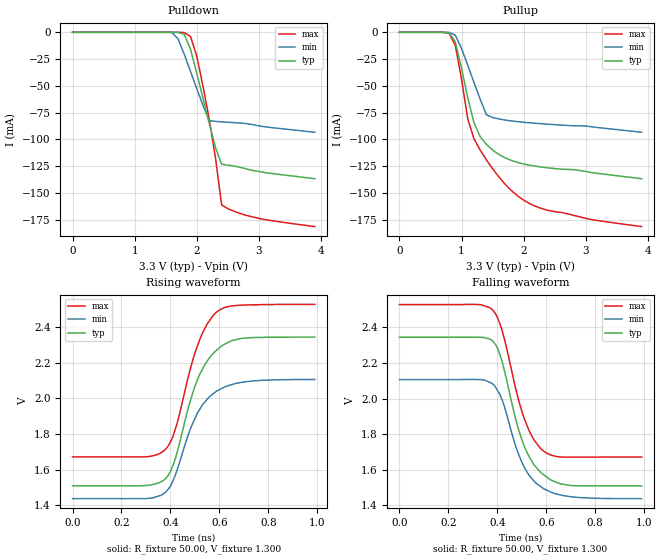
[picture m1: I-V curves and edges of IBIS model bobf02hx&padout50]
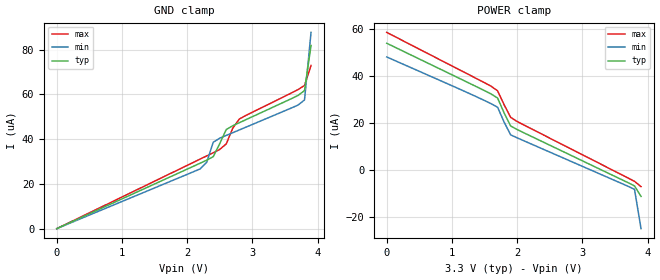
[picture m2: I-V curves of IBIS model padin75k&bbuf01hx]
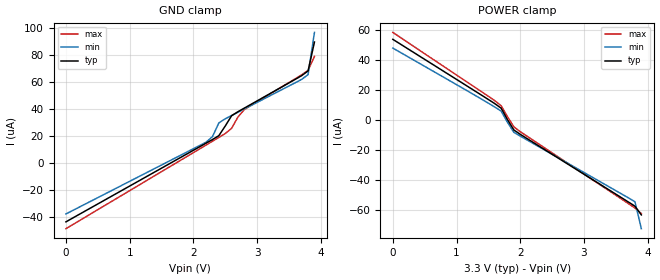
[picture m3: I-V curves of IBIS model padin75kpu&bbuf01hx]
|   This file is an IBIS representation of the   |
|   Integrated Device Technology, Inc.   |
|   MC100ES6254   |
|   2x2 Clock Switch   |
[IBIS Ver]   3.2
[File name]   mc100es6254_3v3.ibs
[File Rev]   0.02
[Date]   7 March 2006 | Last modified
|   7 March 2006 | Generated
[Source]   Originated at Integrated Device Technology, Inc.
[Disclaimer]
   (C) Copyright Integrated Device Technology, Inc. 2005
   All rights reserved
   IDT hereby grants the user of this IBIS model a non-exclusive,
   nontransferable license to use this IBIS model under the following terms.
   Before using this IBIS model, the user should read this license.
   If the user does not accept these terms,  the IBIS model should be
   returned to IDT within 30 days.
   The user is granted this license only to use the IBIS model and
   is not granted rights to sell, load, rent, lease or license the IBIS
   model in whole or in part, or in modified form to anyone other than
   user. User may modify the IBIS model to suit its specific
   applications but rights to derivative works and such modifications
   shall belong to IDT.
   This IBIS model is provided on an "AS IS" basis and IDT makes
   absolutely no warranty with respect to the information contained
   herein. IDT DISCLAIMS AND CUSTOMER WAIVES ALL WARRANTIES, EXPRESS
   OR IMPLIED, INCLUDING WARRANTIES OF MERCHANTABILITY OR FITNESS FOR
   A PARTICULAR PURPOSE. The entire risk as to quality and performance
   is with the Customer. ACCORDINGLY, IN NO EVENT SHALL THE COMPANY BE
   LIABLE FOR ANY DAMAGES, WHETHER IN CONTRACT OR TORT,INCLUDING ANY
   LOST PROFITS OR OTHER INCIDENTAL, CONSEQUENTIAL, EXEMPLARY, OR
   PUNITIVE DAMAGES ARISING OUT OF THE USE OR APPLICATION OF THE IBIS
   model provided in this package. Further, IDT reserves the right to
   make changes without notice to any product herein to improve
   reliability, function, or design. IDT does not convey any license
   under patent rights or any other intellectual property rights,
   including those of third parties.
   IDT is not obligated to provide maintenance or support
   for the licensed IBIS model.
[Copyright]   Copyright 2002 by Integrated Device Technology, Inc.
[Component]   32ld_LQFP
[Manufacturer]   Integrated Device Technology, Inc.
[Package]
   |LQFP32
   |   typ   min   max
   R_pkg   220.4m   212.5m   238m
   L_pkg   1.841n   1.708n   1.974n
   C_pkg   0.316p   0.2907p   0.33p
[Pin]   signal_name   model_name
   1   VCC   POWER
   2   GND   GND
   3   SEL1   padin75k&bc2p01ll
   4   CLK1   padin75k&bbuf01hx
   5   nCLK1   padin75kpu&bbuf01hx
   6   OEB   padin75k&bc2p01ll
   7   GND   GND
   8   VCC   POWER
   9   nQB0   bobf02hx&padout50
   10   QB0   bobf02hx&padout50
   11   VCC   POWER
   12   nQB1   bobf02hx&padout50
   13   QB1   bobf02hx&padout50
   14   VCC   POWER
   15   nQB2   bobf02hx&padout50
   16   QB2   bobf02hx&padout50
   17   VCC   POWER
   18   GND   GND
   19   SEL0   padin75k&bc2p01ll
   20   nCLK0   padin75kpu&bbuf01hx
   21   CLK0   padin75k&bbuf01hx
   22   OEB   padin75k&bc2p01ll
   23   GND   GND
   24   VCC   POWER
   25   QA2   bobf02hx&padout50
   26   nQA2   bobf02hx&padout50
   27   VCC   POWER
   28   QA1   bobf02hx&padout50
   29   nQA1   bobf02hx&padout50
   30   VCC   POWER
   31   QA0   bobf02hx&padout50
   32   nQA0   bobf02hx&padout50
[Diff Pin]   inv_pin  vdiff tdelay_typ tdelay_min  tdelay_max
   4   5   0.0   0   0   0
   21   20   0.0   0   0   0
   31   32   NA   0   0   0
   28   29   NA   0   0   0
   25   26   NA   0   0   0
   16   15   NA   0   0   0
   13   12   NA   0   0   0
   10   9   NA   0   0   0
| Models and submodels in the file (4): bobf02hx&padout50 (Output_ECL), padin75k&bbuf01hx (Input), padin75kpu&bbuf01hx (Input), padin75k&bc2p01ll (Input)
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[Model]   bobf02hx&padout50
   Model_type  Output_ECL
   Polarity   Non-Inverting
   C_comp   1.0p   0.5p   1.5p
   Vmeas =   2.0
   Rref =   50.0
   Cref =   0.0
   Vref =   1.3
[Temperature range]   25.0   -40.0   85.0
[Voltage Range]   3.300   3.135   3.465
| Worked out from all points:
|   rising waveform, R_fixture 50.00, V_fixture 1.300: 20-80 % time 113ps typ, 115ps min, 105ps max; typ from 1.51 V to 2.34 V
|   falling waveform, R_fixture 50.00, V_fixture 1.300: 20-80 % time 104ps typ, 104ps min, 98.4ps max; typ from 2.34 V to 1.51 V
   |  Voltage   I(typ)   I(min)   I(max)
[Pullup]
0V        306fA      113.8fA    11.76pA
800mV     -461.3uA   -42.72uA   -1.009mA
900mV     -8.995mA   -2.712mA   -12.22mA
1V        -33.74mA   -15.14mA   -43.69mA
1.1V      -61.01mA   -30.79mA   -80.81mA
1.2V      -84.45mA   -46.77mA   -99.33mA
1.3V      -97.51mA   -62.46mA   -110mA
1.4V      -104.6mA   -76.94mA   -119.1mA
1.6V      -114mA     -80.92mA   -135mA
1.9V      -121.5mA   -83.42mA   -152.7mA
2.4V      -126.7mA   -85.87mA   -166.4mA
3.9V      -136.7mA   -93.4mA    -181.4mA
[Pulldown]|
0V        309fA      115.4fA    11.77pA
1.6V      -1.553uA   -223.5uA   -494.2nA
1.7V      -63.79uA   -6.301mA   -10.85uA
1.8V      -2.095mA   -20.69mA   -234.6uA
1.9V      -16.08mA   -36.69mA   -3.965mA
2V        -38.22mA   -52.69mA   -22.22mA
2.2V      -84.95mA   -82.6mA    -81.15mA
2.3V      -107.4mA   -83.21mA   -116.8mA
2.4V      -123.2mA   -83.65mA   -161.3mA
2.6V      -124.9mA   -84.43mA   -167.3mA
3V        -130.1mA   -87.45mA   -173.9mA
3.9V      -136.8mA   -93.43mA   -181.5mA
[Ramp]
   |   typ   min   max
   dV/dt_r   0.70V/0.2ns   0.60V/0.20ns   0.84V/0.20ns
   dV/dt_f   0.70V/0.2ns   0.60V/0.20ns   0.84V/0.20ns
   R_load =   50.0000
[Rising Waveform]
   R_fixture =   50.00
   V_fixture =   1.300
   V_fixture_min =  1.135
   V_fixture_max =  1.465
| time(s)   voltage(typ)   voltage(min)   voltage(max)
0s        1.51V      1.438V     1.672V
310ps     1.513V     1.44V      1.674V
380ps     1.55V      1.474V     1.714V
420ps     1.662V     1.569V     1.828V
480ps     1.981V     1.823V     2.158V
520ps     2.136V     1.939V     2.33V
550ps     2.209V     1.995V     2.417V
600ps     2.284V     2.049V     2.495V
700ps     2.338V     2.092V     2.523V
990ps     2.344V     2.106V     2.527V
[Falling Waveform]
   R_fixture =   50.00
   V_fixture =   1.300
   V_fixture_min =  1.135
   V_fixture_max =  1.465
|   time(s)   voltage(typ)   voltage(min)   voltage(max)
0s        2.344V     2.106V     2.527V
330ps     2.343V     2.106V     2.527V
380ps     2.324V     2.084V     2.498V
420ps     2.206V     1.992V     2.381V
480ps     1.859V     1.713V     2.03V
510ps     1.733V     1.615V     1.888V
550ps     1.628V     1.537V     1.768V
600ps     1.561V     1.487V     1.695V
700ps     1.512V     1.449V     1.671V
990ps     1.51V      1.438V     1.672V
|..............................................................................|
| .  .  .  .  .  .  .  .  .  .  .  .  .  .  .  .  .  .  .  .  .  .  .  .  .  . |
|..............................................................................|
[Model]   padin75k&bbuf01hx
   Model_type   Input
   Polarity   Non-Inverting
   Vinl =   0.6V
   Vinh =   0.9V
   C_comp   1.0p   0.5p   1.5p
[Temperature range]   25.0   -40.0   85.0
[Voltage Range]   3.300   3.135   3.465
   |  Voltage   I(typ)   I(min)   I(max)
[GND_clamp]
|   -3.3000e+00   -7.9104e+04   -9.9835e+04   -6.6693e+04
|   -3.2000e+00   -7.5545e+04   -9.5284e+04   -6.3730e+04
|   -3.1000e+00   -7.1986e+04   -9.0733e+04   -6.0767e+04
|   -3.0000e+00   -6.8428e+04   -8.6182e+04   -5.7805e+04
|   -2.9000e+00   -6.4869e+04   -8.1632e+04   -5.4842e+04
|   -2.8000e+00   -6.1310e+04   -7.7081e+04   -5.1880e+04
|   -2.7000e+00   -5.7751e+04   -7.2530e+04   -4.8917e+04
|   -2.6000e+00   -5.4192e+04   -6.7979e+04   -4.5954e+04
|   -2.5000e+00   -5.0634e+04   -6.3428e+04   -4.2992e+04
|   -2.4000e+00   -4.7075e+04   -5.8877e+04   -4.0029e+04
|   -2.3000e+00   -4.3516e+04   -5.4326e+04   -3.7067e+04
|   -2.2000e+00   -3.9957e+04   -4.9775e+04   -3.4104e+04
|   -2.1000e+00   -3.6398e+04   -4.5224e+04   -3.1141e+04
|   -2.0000e+00   -3.2840e+04   -4.0673e+04   -2.8179e+04
|   -1.9000e+00   -2.9281e+04   -3.6122e+04   -2.5216e+04
|   -1.8000e+00   -2.5722e+04   -3.1571e+04   -2.2254e+04
|   -1.7000e+00   -2.2163e+04   -2.7020e+04   -1.9291e+04
|   -1.6000e+00   -1.8604e+04   -2.2469e+04   -1.6328e+04
|   -1.5000e+00   -1.5046e+04   -1.7918e+04   -1.3366e+04
|   -1.4000e+00   -1.1487e+04   -1.3367e+04   -1.0403e+04
|   -1.3000e+00   -7.9281e+03   -8.8163e+03   -7.4406e+03
|   -1.2000e+00   -4.3693e+03   -4.2653e+03   -4.4780e+03
|   -1.1000e+00   -8.7191e+02   -2.7260e+02   -1.5154e+03
|   -1.0000e+00   -1.8440e+01   -1.8787e+00   -7.6527e+01
|   -9.0000e-01   -3.7617e-01   -1.2959e-02   -2.9964e+00
|   -8.0000e-01   -7.6837e-03   -9.8936e-05   -1.1734e-01
|   -7.0000e-01   -1.6583e-04   -9.1041e-06   -4.6038e-03
|   -6.0000e-01   -1.1170e-05   -7.2806e-06   -1.8835e-04
|   -5.0000e-01   -6.7130e-06   -6.0637e-06   -1.4108e-05
|   -4.0000e-01   -5.3196e-06   -4.8509e-06   -5.9277e-06
|   -3.0000e-01   -3.9888e-06   -3.6382e-06   -4.2497e-06
|   -2.0000e-01   -2.6592e-06   -2.4255e-06   -2.8264e-06
|   -1.0000e-01   -1.3296e-06   -1.2127e-06   -1.4130e-06
0V        -252.6fA   -122.9fA   -7.579pA
2.2V      29.25uA    26.7uA     31.08uA
2.3V      30.59uA    29.63uA    32.5uA
2.4V      32.17uA    38.6uA     33.91uA
2.5V      38uA       40.42uA    35.38uA
2.6V      44.32uA    41.65uA    37.88uA
2.7V      45.98uA    42.88uA    44.91uA
2.8V      47.33uA    44.1uA     48.97uA
3.7V      59.49uA    55.18uA    62.11uA
3.8V      61.67uA    57.51uA    63.98uA
3.9V      81.81uA    87.68uA    72.92uA
|   4.0000e+00   2.0121e-04   5.3891e-04   1.3526e-04
|   4.1000e+00   1.4710e-03   4.7993e-02   3.6059e-04
|   4.2000e+00   5.4971e-02   6.9042e+00   2.5491e-03
|   4.3000e+00   2.6670e+00   9.9777e+02   5.3444e-02
|   4.4000e+00   1.3071e+02   5.5487e+03   1.3476e+00
|   4.5000e+00   2.6945e+03   1.0100e+04   3.4394e+01
|   4.6000e+00   6.2533e+03   1.4651e+04   8.7836e+02
|   4.7000e+00   9.8121e+03   1.9202e+04   3.8402e+03
|   4.8000e+00   1.3371e+04   2.3753e+04   6.8028e+03
|   4.9000e+00   1.6930e+04   2.8303e+04   9.7654e+03
|   5.0000e+00   2.0489e+04   3.2854e+04   1.2728e+04
|   5.1000e+00   2.4047e+04   3.7405e+04   1.5691e+04
|   5.2000e+00   2.7606e+04   4.1956e+04   1.8653e+04
|   5.3000e+00   3.1165e+04   4.6507e+04   2.1616e+04
|   5.4000e+00   3.4724e+04   5.1058e+04   2.4578e+04
|   5.5000e+00   3.8282e+04   5.5609e+04   2.7541e+04
|   5.6000e+00   4.1841e+04   6.0160e+04   3.0504e+04
|   5.7000e+00   4.5400e+04   6.4711e+04   3.3466e+04
|   5.8000e+00   4.8959e+04   6.9262e+04   3.6429e+04
|   5.9000e+00   5.2518e+04   7.3813e+04   3.9391e+04
|   6.0000e+00   5.6076e+04   7.8364e+04   4.2354e+04
|   6.1000e+00   5.9635e+04   8.2915e+04   4.5317e+04
|   6.2000e+00   6.3194e+04   8.7466e+04   4.8279e+04
|   6.3000e+00   6.6753e+04   9.2017e+04   5.1242e+04
|   6.4000e+00   7.0312e+04   9.6568e+04   5.4204e+04
|   6.5000e+00   7.3870e+04   1.0112e+05   5.7167e+04
|   6.6000e+00   7.7429e+04   1.0567e+05   6.0130e+04
[POWER_clamp]
|   -3.3000e+00   7.7429e+04   9.8161e+04   6.5018e+04
|   -3.2000e+00   7.3870e+04   9.3610e+04   6.2055e+04
|   -3.1000e+00   7.0312e+04   8.9059e+04   5.9093e+04
|   -3.0000e+00   6.6753e+04   8.4508e+04   5.6130e+04
|   -2.9000e+00   6.3194e+04   7.9957e+04   5.3168e+04
|   -2.8000e+00   5.9635e+04   7.5406e+04   5.0205e+04
|   -2.7000e+00   5.6076e+04   7.0855e+04   4.7242e+04
|   -2.6000e+00   5.2518e+04   6.6304e+04   4.4280e+04
|   -2.5000e+00   4.8959e+04   6.1753e+04   4.1317e+04
|   -2.4000e+00   4.5400e+04   5.7202e+04   3.8355e+04
|   -2.3000e+00   4.1841e+04   5.2651e+04   3.5392e+04
|   -2.2000e+00   3.8282e+04   4.8100e+04   3.2429e+04
|   -2.1000e+00   3.4724e+04   4.3549e+04   2.9467e+04
|   -2.0000e+00   3.1165e+04   3.8998e+04   2.6504e+04
|   -1.9000e+00   2.7606e+04   3.4447e+04   2.3542e+04
|   -1.8000e+00   2.4047e+04   2.9896e+04   2.0579e+04
|   -1.7000e+00   2.0489e+04   2.5345e+04   1.7616e+04
|   -1.6000e+00   1.6930e+04   2.0794e+04   1.4654e+04
|   -1.5000e+00   1.3371e+04   1.6243e+04   1.1691e+04
|   -1.4000e+00   9.8121e+03   1.1693e+04   8.7285e+03
|   -1.3000e+00   6.2533e+03   7.1416e+03   5.7659e+03
|   -1.2000e+00   2.6945e+03   2.5906e+03   2.8033e+03
|   -1.1000e+00   1.3071e+02   3.9415e+01   2.8259e+02
|   -1.0000e+00   2.6670e+00   2.7213e-01   1.1066e+01
|   -9.0000e-01   5.4971e-02   2.1495e-03   4.3412e-01
|   -8.0000e-01   1.4712e-03   1.2845e-04   1.7596e-02
|   -7.0000e-01   2.0125e-04   6.1367e-05   1.0731e-03
|   -6.0000e-01   8.1825e-05   5.5665e-05   2.4548e-04
|   -5.0000e-01   6.1679e-05   5.4364e-05   1.0249e-04
|   -4.0000e-01   5.9491e-05   5.3123e-05   6.7451e-05
|   -3.0000e-01   5.8099e-05   5.1890e-05   6.3195e-05
|   -2.0000e-01   5.6742e-05   5.0659e-05   6.1579e-05
|   -1.0000e-01   5.5392e-05   4.9431e-05   6.0108e-05
0V        54.05uA    48.2uA     58.67uA
1.5V      33.85uA    29.65uA    37.23uA
1.6V      32.45uA    28.31uA    35.77uA
1.7V      30.72uA    26.8uA     33.79uA
1.8V      24.4uA     20.48uA    27.85uA
1.9V      18.83uA    15.06uA    22.5uA
2V        17.29uA    13.76uA    20.72uA
3.8V      -6.713uA   -8.172uA   -4.767uA
3.9V      -11.17uA   -24.91uA   -7.004uA
|   4.0000e+00   -1.6583e-04   -2.2783e-03   -2.9451e-05
|   4.1000e+00   -7.6837e-03   -3.2907e-01   -5.6808e-04
|   4.2000e+00   -3.7617e-01   -4.7747e+01   -1.4290e-02
|   4.3000e+00   -1.8440e+01   -2.6725e+03   -3.6469e-01
|   4.4000e+00   -8.7191e+02   -7.2234e+03   -9.3138e+00
|   4.5000e+00   -4.3693e+03   -1.1774e+04   -2.3787e+02
|   4.6000e+00   -7.9281e+03   -1.6325e+04   -2.5524e+03
|   4.7000e+00   -1.1487e+04   -2.0876e+04   -5.5150e+03
|   4.8000e+00   -1.5046e+04   -2.5427e+04   -8.4775e+03
|   4.9000e+00   -1.8604e+04   -2.9978e+04   -1.1440e+04
|   5.0000e+00   -2.2163e+04   -3.4529e+04   -1.4403e+04
|   5.1000e+00   -2.5722e+04   -3.9080e+04   -1.7365e+04
|   5.2000e+00   -2.9281e+04   -4.3631e+04   -2.0328e+04
|   5.3000e+00   -3.2840e+04   -4.8182e+04   -2.3291e+04
|   5.4000e+00   -3.6398e+04   -5.2733e+04   -2.6253e+04
|   5.5000e+00   -3.9957e+04   -5.7284e+04   -2.9216e+04
|   5.6000e+00   -4.3516e+04   -6.1835e+04   -3.2178e+04
|   5.7000e+00   -4.7075e+04   -6.6386e+04   -3.5141e+04
|   5.8000e+00   -5.0634e+04   -7.0937e+04   -3.8104e+04
|   5.9000e+00   -5.4192e+04   -7.5488e+04   -4.1066e+04
|   6.0000e+00   -5.7751e+04   -8.0039e+04   -4.4029e+04
|   6.1000e+00   -6.1310e+04   -8.4590e+04   -4.6991e+04
|   6.2000e+00   -6.4869e+04   -8.9141e+04   -4.9954e+04
|   6.3000e+00   -6.8428e+04   -9.3692e+04   -5.2917e+04
|   6.4000e+00   -7.1986e+04   -9.8242e+04   -5.5879e+04
|   6.5000e+00   -7.5545e+04   -1.0279e+05   -5.8842e+04
|   6.6000e+00   -7.9104e+04   -1.0734e+05   -6.1804e+04
|..............................................................................|
| .  .  .  .  .  .  .  .  .  .  .  .  .  .  .  .  .  .  .  .  .  .  .  .  .  . |
|..............................................................................|
[Model]   padin75kpu&bbuf01hx
   Model_type   Input
   Polarity   Non-Inverting
   Vinl =   0.6V
   Vinh =   0.9V
   C_comp   1.0p   0.5p   1.5p
[Temperature range]   25.0   -40.0   85.0
[Voltage Range]   3.300   3.135   3.465
   |  Voltage   I(typ)   I(min)   I(max)
[GND_clamp]
|   -3.3000e+00   -7.9104e+04   -9.9835e+04   -6.6693e+04
|   -3.2000e+00   -7.5545e+04   -9.5284e+04   -6.3730e+04
|   -3.1000e+00   -7.1986e+04   -9.0733e+04   -6.0767e+04
|   -3.0000e+00   -6.8428e+04   -8.6182e+04   -5.7805e+04
|   -2.9000e+00   -6.4869e+04   -8.1632e+04   -5.4842e+04
|   -2.8000e+00   -6.1310e+04   -7.7081e+04   -5.1880e+04
|   -2.7000e+00   -5.7751e+04   -7.2530e+04   -4.8917e+04
|   -2.6000e+00   -5.4192e+04   -6.7979e+04   -4.5954e+04
|   -2.5000e+00   -5.0634e+04   -6.3428e+04   -4.2992e+04
|   -2.4000e+00   -4.7075e+04   -5.8877e+04   -4.0029e+04
|   -2.3000e+00   -4.3516e+04   -5.4326e+04   -3.7067e+04
|   -2.2000e+00   -3.9957e+04   -4.9775e+04   -3.4104e+04
|   -2.1000e+00   -3.6398e+04   -4.5224e+04   -3.1141e+04
|   -2.0000e+00   -3.2840e+04   -4.0673e+04   -2.8179e+04
|   -1.9000e+00   -2.9281e+04   -3.6122e+04   -2.5216e+04
|   -1.8000e+00   -2.5722e+04   -3.1571e+04   -2.2254e+04
|   -1.7000e+00   -2.2163e+04   -2.7020e+04   -1.9291e+04
|   -1.6000e+00   -1.8604e+04   -2.2469e+04   -1.6328e+04
|   -1.5000e+00   -1.5046e+04   -1.7918e+04   -1.3366e+04
|   -1.4000e+00   -1.1487e+04   -1.3367e+04   -1.0403e+04
|   -1.3000e+00   -7.9281e+03   -8.8163e+03   -7.4406e+03
|   -1.2000e+00   -4.3693e+03   -4.2653e+03   -4.4780e+03
|   -1.1000e+00   -8.7191e+02   -2.7260e+02   -1.5154e+03
|   -1.0000e+00   -1.8440e+01   -1.8788e+00   -7.6527e+01
|   -9.0000e-01   -3.7622e-01   -1.3008e-02   -2.9965e+00
|   -8.0000e-01   -7.7382e-03   -1.4666e-04   -1.1740e-01
|   -7.0000e-01   -2.1901e-04   -5.5612e-05   -4.6626e-03
|   -6.0000e-01   -6.3024e-05   -5.2576e-05   -2.4579e-04
|   -5.0000e-01   -5.7237e-05   -5.0146e-05   -7.0132e-05
|   -4.0000e-01   -5.4514e-05   -4.7721e-05   -6.0539e-05
|   -3.0000e-01   -5.1854e-05   -4.5295e-05   -5.7448e-05
|   -2.0000e-01   -4.9194e-05   -4.2870e-05   -5.4612e-05
|   -1.0000e-01   -4.6535e-05   -4.0444e-05   -5.1785e-05
0V        -43.88uA   -38.02uA   -48.96uA
2.2V      14.63uA    15.36uA    13.21uA
2.3V      17.29uA    19.51uA    16.04uA
2.4V      20.2uA     29.69uA    18.87uA
2.5V      27.36uA    32.72uA    21.75uA
2.6V      35.01uA    35.16uA    25.66uA
2.7V      38uA       37.6uA     34.1uA
2.8V      40.68uA    40.04uA    39.57uA
3.7V      64.81uA    62.03uA    65.43uA
3.8V      68.32uA    65.57uA    68.71uA
3.9V      89.79uA    96.95uA    79.07uA
|   4.0000e+00   2.1052e-04   5.4940e-04   1.4282e-04
|   4.1000e+00   1.4817e-03   4.8005e-02   3.6957e-04
|   4.2000e+00   5.4983e-02   6.9042e+00   2.5594e-03
|   4.3000e+00   2.6670e+00   9.9777e+02   5.3456e-02
|   4.4000e+00   1.3071e+02   5.5487e+03   1.3476e+00
|   4.5000e+00   2.6945e+03   1.0100e+04   3.4394e+01
|   4.6000e+00   6.2533e+03   1.4651e+04   8.7836e+02
|   4.7000e+00   9.8121e+03   1.9202e+04   3.8402e+03
|   4.8000e+00   1.3371e+04   2.3753e+04   6.8028e+03
|   4.9000e+00   1.6930e+04   2.8303e+04   9.7654e+03
|   5.0000e+00   2.0489e+04   3.2854e+04   1.2728e+04
|   5.1000e+00   2.4047e+04   3.7405e+04   1.5691e+04
|   5.2000e+00   2.7606e+04   4.1956e+04   1.8653e+04
|   5.3000e+00   3.1165e+04   4.6507e+04   2.1616e+04
|   5.4000e+00   3.4724e+04   5.1058e+04   2.4578e+04
|   5.5000e+00   3.8282e+04   5.5609e+04   2.7541e+04
|   5.6000e+00   4.1841e+04   6.0160e+04   3.0504e+04
|   5.7000e+00   4.5400e+04   6.4711e+04   3.3466e+04
|   5.8000e+00   4.8959e+04   6.9262e+04   3.6429e+04
|   5.9000e+00   5.2518e+04   7.3813e+04   3.9391e+04
|   6.0000e+00   5.6076e+04   7.8364e+04   4.2354e+04
|   6.1000e+00   5.9635e+04   8.2915e+04   4.5317e+04
|   6.2000e+00   6.3194e+04   8.7466e+04   4.8279e+04
|   6.3000e+00   6.6753e+04   9.2017e+04   5.1242e+04
|   6.4000e+00   7.0312e+04   9.6568e+04   5.4204e+04
|   6.5000e+00   7.3870e+04   1.0112e+05   5.7167e+04
|   6.6000e+00   7.7429e+04   1.0567e+05   6.0130e+04
[POWER_clamp]
|   -3.3000e+00   7.7429e+04   9.8161e+04   6.5018e+04
|   -3.2000e+00   7.3870e+04   9.3610e+04   6.2055e+04
|   -3.1000e+00   7.0312e+04   8.9059e+04   5.9093e+04
|   -3.0000e+00   6.6753e+04   8.4508e+04   5.6130e+04
|   -2.9000e+00   6.3194e+04   7.9957e+04   5.3168e+04
|   -2.8000e+00   5.9635e+04   7.5406e+04   5.0205e+04
|   -2.7000e+00   5.6076e+04   7.0855e+04   4.7242e+04
|   -2.6000e+00   5.2518e+04   6.6304e+04   4.4280e+04
|   -2.5000e+00   4.8959e+04   6.1753e+04   4.1317e+04
|   -2.4000e+00   4.5400e+04   5.7202e+04   3.8355e+04
|   -2.3000e+00   4.1841e+04   5.2651e+04   3.5392e+04
|   -2.2000e+00   3.8282e+04   4.8100e+04   3.2429e+04
|   -2.1000e+00   3.4724e+04   4.3549e+04   2.9467e+04
|   -2.0000e+00   3.1165e+04   3.8998e+04   2.6504e+04
|   -1.9000e+00   2.7606e+04   3.4447e+04   2.3542e+04
|   -1.8000e+00   2.4047e+04   2.9896e+04   2.0579e+04
|   -1.7000e+00   2.0489e+04   2.5345e+04   1.7616e+04
|   -1.6000e+00   1.6930e+04   2.0794e+04   1.4654e+04
|   -1.5000e+00   1.3371e+04   1.6243e+04   1.1691e+04
|   -1.4000e+00   9.8121e+03   1.1693e+04   8.7285e+03
|   -1.3000e+00   6.2533e+03   7.1416e+03   5.7659e+03
|   -1.2000e+00   2.6945e+03   2.5906e+03   2.8033e+03
|   -1.1000e+00   1.3071e+02   3.9415e+01   2.8259e+02
|   -1.0000e+00   2.6670e+00   2.7214e-01   1.1066e+01
|   -9.0000e-01   5.4983e-02   2.1604e-03   4.3413e-01
|   -8.0000e-01   1.4818e-03   1.3815e-04   1.7608e-02
|   -7.0000e-01   2.1056e-04   6.9856e-05   1.0830e-03
|   -6.0000e-01   8.9803e-05   6.2941e-05   2.5396e-04
|   -5.0000e-01   6.8327e-05   6.0427e-05   1.0956e-04
|   -4.0000e-01   6.4810e-05   5.7974e-05   7.3103e-05
|   -3.0000e-01   6.2088e-05   5.5528e-05   6.7434e-05
|   -2.0000e-01   5.9401e-05   5.3085e-05   6.4405e-05
|   -1.0000e-01   5.6722e-05   5.0644e-05   6.1521e-05
0V        54.05uA    48.2uA     58.67uA
1.5V      13.9uA     11.46uA    16.04uA
1.7V      8.117uA    6.186uA    9.767uA
1.8V      466.4nA    -1.35uA    2.414uA
1.9V      -6.428uA   -7.985uA   -4.344uA
3.8V      -57.24uA   -54.26uA   -58.46uA
3.9V      -63.02uA   -72.2uA    -62.11uA
